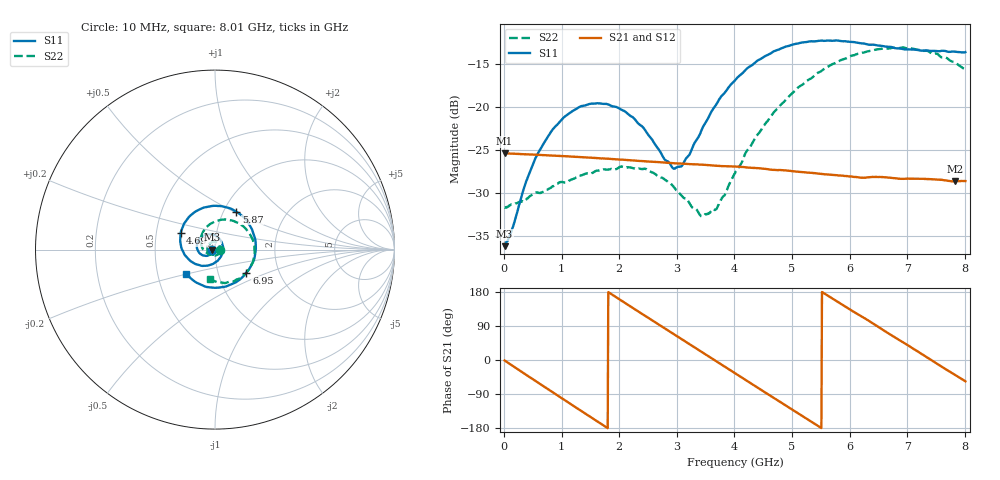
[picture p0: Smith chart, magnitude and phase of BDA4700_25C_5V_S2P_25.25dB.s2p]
!Agilent Technologies,E5071B,MY42404982,A.09.10
!Date: Mon Oct 20 13:39:11 2025
!Data & Calibration Information:
!Freq	S11:SOLT2(ON)	S21:SOLT2(ON)	S12:SOLT2(ON)	S22:SOLT2(ON)
# Hz S RI R 50
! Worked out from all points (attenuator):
!   801 points, 10 MHz to 8.01 GHz, reference 50 ohm
!   highest |S21| = -25.32 dB at 10 MHz (marker M1); lowest = -28.6 dB at 7.83 GHz (marker M2)
!   lowest |S11| = -36.1 dB at 10 MHz (marker M3), VSWR 1.03, Z = 48.5 - j0.122 ohm
!   |S11| at or under -10 dB: start of sweep to end of sweep
!   |S22| runs from -32.7 to -13.0 dB; largest |S21 - S12| = 0.00042
!   S11 on the Smith chart (normalised r, x): 10 MHz: 0.97, -0.00; 4.69 GHz: 0.67, +0.13; 5.87 GHz: 1.14, +0.52; 6.95 GHz: 1.37, -0.37; 8.01 GHz: 0.70, -0.20
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1e7  -0.0155 -0.00126  0.0542 -0.00117  0.0541 -0.00122  0.0261 -0.000836
1.2e8  -0.0165 -0.00855  0.0525 -0.0116  0.0525 -0.0116  0.0265 -0.00578
3.7e8  -0.0256 -0.025  0.0423 -0.0326  0.0422 -0.0326  0.0216 -0.019
6e8  -0.0426 -0.0346  0.0259 -0.0461  0.0259 -0.0462  0.0128 -0.0291
1e9  -0.0814 -0.0238  -0.00957 -0.0512  -0.00956 -0.0512  -0.0146 -0.0338
1.35e9  -0.1011 0.0118  -0.0365 -0.036  -0.0365 -0.036  -0.0361 -0.0178
2.07e9  -0.0449 0.0846  -0.0444 0.0221  -0.0444 0.022  -0.0305 0.0333
2.68e9  0.0353 0.0451  -0.00342 0.0479  -0.00342 0.0479  0.0129 0.0373
2.93e9  0.0441 0.00434  0.0163 0.0444  0.0163 0.0444  0.0248 0.0246
3.06e9  0.0413 -0.0184  0.0255 0.0396  0.0253 0.0397  0.0275 0.0147
3.44e9  -0.00347 -0.0751  0.0435 0.0163  0.0435 0.0163  0.0185 -0.0142
3.69e9  -0.0535 -0.0899  0.0457 -0.00283  0.0457 -0.00295  0.000522 -0.0256
4.01e9  -0.1246 -0.0711  0.0373 -0.0256  0.0373 -0.0256  -0.0323 -0.0258
4.69e9  -0.1918 0.0906  -0.00794 -0.0425  -0.00788 -0.0426  -0.08 0.0494
5.35e9  -0.0556 0.2354  -0.04 -0.0112  -0.04 -0.0113  -0.0155 0.148
5.87e9  0.1178 0.2121  -0.0333 0.0223  -0.0332 0.0222  0.1004 0.1605
6.26e9  0.2073 0.1093  -0.0135 0.0366  -0.0131 0.0367  0.1814 0.1037
6.68e9  0.2211 -0.0417  0.0136 0.0366  0.0136 0.0366  0.22 -2.11e-05
6.95e9  0.1754 -0.1281  0.0274 0.027  0.0275 0.0269  0.2096 -0.0735
7.38e9  0.0431 -0.2091  0.0382 0.00233  0.0382 0.00221  0.1344 -0.1619
7.83e9  -0.1142 -0.1772  0.0288 -0.0233  0.0288 -0.0233  0.013 -0.1818
8.01e9  -0.1612 -0.1337  0.0207 -0.031  0.0208 -0.0309  -0.0306 -0.1619
